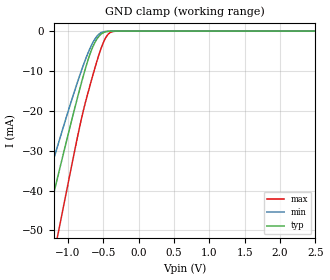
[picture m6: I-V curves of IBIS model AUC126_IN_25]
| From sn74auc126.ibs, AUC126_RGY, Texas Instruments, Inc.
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[Model]   AUC126_IN_25
Model_type  Input
Vinl=0.7
Vinh=1.7
| variable   typ   min   max
C_comp   2.25pF   1.81pF   2.68pF
[Temperature Range]   40   100   -40
| Ambient temperature   25   85   -40
[Voltage range]   2.5   2.3   2.7
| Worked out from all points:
|   GND clamp passes 1 mA (typ) near -0.55 V on its own axis
[GND Clamp]
| AUC126_IN_25
|   Voltage   I(typ)   I(min)   I(max)
-3.6V     -222.3mA   -186mA     -267.4mA
-1.49V    -62.27mA   -49.76mA   -82.08mA
-1.35V    -51.78mA   -41.12mA   -69.61mA
-1.305V   -48.43mA   -38.37mA   -65.59mA
-1.17V    -38.45mA   -30.23mA   -53.54mA
-1.12V    -34.78mA   -27.27mA   -49.07mA
-735mV    -8.323mA   -6.326mA   -16.67mA
-635mV    -3.426mA   -2.469mA   -10.25mA
-525mV    -682.5uA   -360.1uA   -4.021mA
-430mV    -73.19uA   -34.72uA   -776.9uA
-325mV    -3.339uA   -2.005uA   -30.74uA
2.5V      313.9pA    400.8pA    470.4pA
